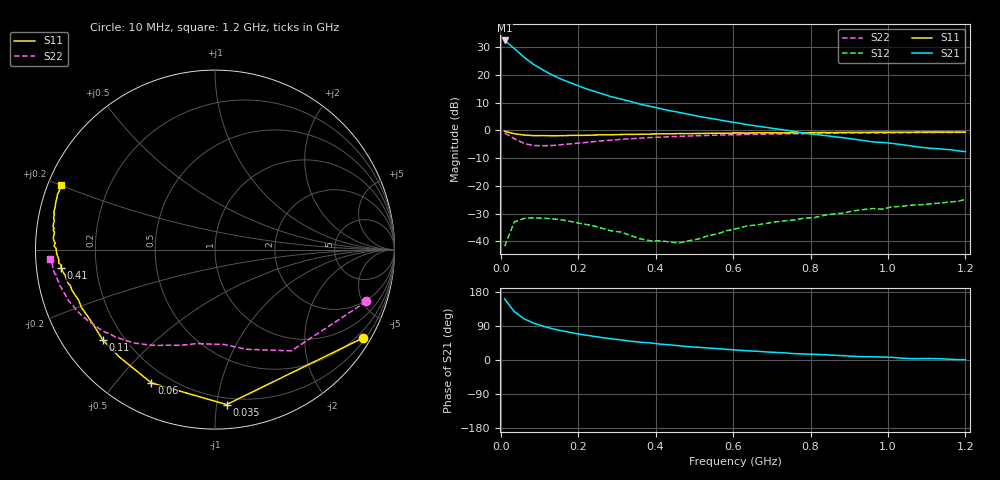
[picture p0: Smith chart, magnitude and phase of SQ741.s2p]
!  POLYFET RF DEVICES
!  SQ741 (EACH SIDE)
!  S PARAMETERS
!  VDS=50V, IDQ=200mA
# MHZ S MA R 50
! Freq=Mhz Mag[s11] Ang[s11] Mag[s21] Ang[s21] Mag[s12] Ang[s12] Mag[s22] Ang[s22]
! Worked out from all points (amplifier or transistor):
!   49 points, 10 MHz to 1.2 GHz, reference 50 ohm
!   highest |S21| = 32.4 dB at 10 MHz (marker M1)
!   |S21| within 3 dB of that: start of sweep to 35.84 MHz
!   unconditionally stable (mu >= 1): 321.7 MHz to 758.1 MHz; 765.1 MHz to 812.5 MHz
!   at 210 MHz: K = 0.52, MSG = 24.6 dB, |S12| = -33.7 dB
!   at 610 MHz: K = 1.21, MAG = 16.3 dB, |S12| = -35.4 dB
!   at 1.2 GHz: K = 0.79, MSG = 8.6 dB, |S12| = -24.8 dB
!   S11 on the Smith chart (normalised r, x): 10 MHz: 0.28, -3.61; 35 MHz: 0.15, -1.07; 60 MHz: 0.14, -0.62; 110 MHz: 0.12, -0.35; 410 MHz: 0.07, -0.06; 1.2 GHz: 0.04, +0.20
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10  0.9607 -30.8  41.47 161.3  0.00819 68.6  0.892 -18.9
35  0.8657 -85.7  29.72 127.7  0.02228 40.8  0.7064 -53.0
60  0.823 -115.5  20.82 108.8  0.0259 21.7  0.5815 -72.7
85  0.8011 -131.7  15.33 97.2  0.02657 13.0  0.531 -84.5
110  0.8027 -141.3  12.09 89.2  0.02608 6.7  0.5275 -93.6
135  0.7964 -148.0  9.736 82.1  0.02546 0.5  0.5328 -100.8
160  0.8006 -152.4  8.13 76.7  0.0242 -0.2  0.5526 -106.5
185  0.8111 -156.6  6.954 71.6  0.02254 -5.2  0.5737 -111.6
210  0.8103 -159.6  5.943 67.0  0.02068 -6.6  0.5946 -116.4
235  0.8183 -161.7  5.205 63.3  0.01939 -6.7  0.6197 -120.5
260  0.8291 -164.3  4.588 59.4  0.01735 -5.4  0.6446 -124.3
285  0.8303 -165.9  4.039 56.1  0.01547 -6.0  0.664 -127.7
335  0.8448 -169.1  3.305 49.8  0.01275 2.3  0.7039 -133.6
360  0.8474 -170.3  2.955 47.0  0.01115 8.8  0.7213 -136.4
410  0.8628 -173.2  2.482 42.1  0.01021 25.1  0.7499 -141.3
460  0.8737 -175.1  2.107 37.7  0.00934 38.8  0.7771 -145.0
485  0.8724 -176.5  1.94 35.1  0.01022 54.1  0.7898 -147.2
610  0.8972 178.8  1.365 26.3  0.01701 80.7  0.8325 -154.7
685  0.9034 176.0  1.129 21.4  0.02097 82.3  0.8522 -158.8
810  0.9104 172.1  0.8471 15.1  0.02674 90.7  0.8757 -164.3
1010  0.9213 165.1  0.5819 6.9  0.04187 93.7  0.9026 -171.5
1200  0.9288 157.3  0.4127 0.7  0.0573 91.9  0.9181 -176.8
